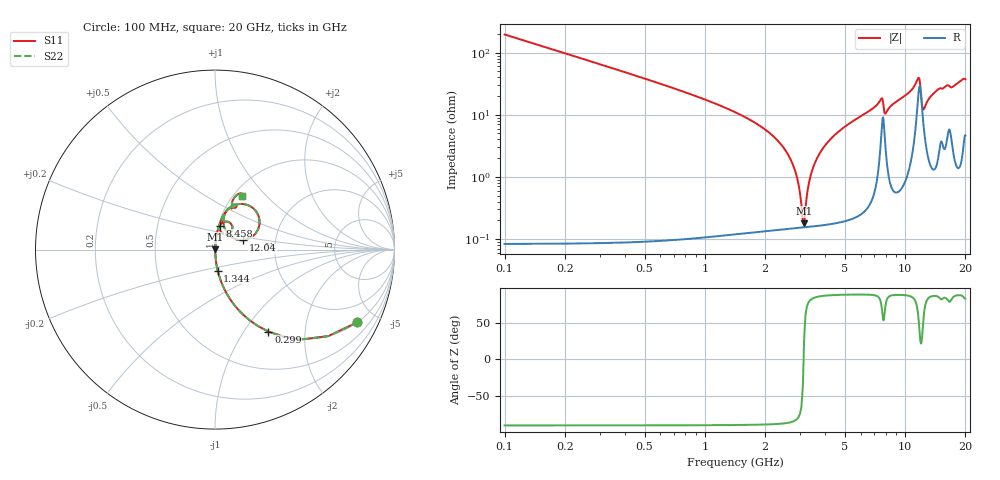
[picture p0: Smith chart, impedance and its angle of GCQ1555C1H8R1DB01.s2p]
!Murata Part Number: GCQ1555C1H8R1DB01
!These Parameters are Measured in Series Mode Connection
!Data Generated on Jan 08, 2026
!  o--ll--o
!Port1  Port2
!  o------o
!Operation Temp=25[degC], DC Bias Voltage=0[V]
!Freq. Start=100[MHz] Stop=20[GHz] 401[Steps]
# Hz S RI R 50
!Freq.(Hz) S11(Real) S11(Imag) S21(Real) S21(Imag) S12(Real) S12(Imag) S22(Real) S22(Imag)
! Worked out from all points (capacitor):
!   401 points, 100 MHz to 20 GHz, reference 50 ohm
!   read as one part in series: C = 8.1 pF near 199.5 MHz
!   lowest |Z| = 178 mohm at 3.135 GHz (marker M1)
!   series resonance near 3.113 GHz, so ESL is about 320 pH
!   S11 on the Smith chart (normalised r, x): 100 MHz: 1.00, -3.93; 299 MHz: 1.00, -1.30; 1.344 GHz: 1.00, -0.24; 8.458 GHz: 1.01, +0.27; 12.04 GHz: 1.37, +0.15; 20 GHz: 1.09, +0.74
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1e8  0.7938 -0.4043  0.2062 0.4043  0.2062 0.4043  0.7938 -0.4043
2.99e8  0.2979 -0.4567  0.7021 0.4567  0.7021 0.4567  0.2979 -0.4567
5.975e8  0.0918 -0.2873  0.9082 0.2873  0.9082 0.2873  0.0918 -0.2873
1.34375e9  0.0151 -0.117  0.9849 0.117  0.9849 0.117  0.0151 -0.117
2.5875e9  0.00199 -0.0235  0.998 0.0235  0.998 0.0235  0.00199 -0.0235
2.83625e9  0.00162 -0.0118  0.9984 0.0118  0.9984 0.0118  0.00162 -0.0118
3.03525e9  0.00152 -0.00319  0.9985 0.00319  0.9985 0.00319  0.00152 -0.00319
3.13475e9  0.00153 0.000904  0.9985 -0.000904  0.9985 -0.000904  0.00153 0.000904
3.43325e9  0.00174 0.0125  0.9983 -0.0125  0.9983 -0.0125  0.00174 0.0125
3.83125e9  0.00236 0.0267  0.9976 -0.0267  0.9976 -0.0267  0.00236 0.0267
4.42825e9  0.00391 0.0462  0.9961 -0.0462  0.9961 -0.0462  0.00391 0.0462
6.7665e9  0.0182 0.1182  0.9818 -0.1182  0.9818 -0.1182  0.0182 0.1182
7.61225e9  0.0736 0.155  0.9264 -0.155  0.9264 -0.155  0.0736 0.155
7.9605e9  0.041 0.0917  0.959 -0.0917  0.959 -0.0917  0.041 0.0917
8.458e9  0.0253 0.1321  0.9747 -0.1321  0.9747 -0.1321  0.0253 0.1321
1.005e10  0.048 0.1936  0.952 -0.1936  0.952 -0.1936  0.048 0.1936
1.159225e10  0.2143 0.229  0.7857 -0.229  0.7857 -0.229  0.2143 0.229
1.204e10  0.1585 0.053  0.8415 -0.053  0.8415 -0.053  0.1585 0.053
1.23385e10  0.0744 0.0849  0.9256 -0.0849  0.9256 -0.0849  0.0744 0.0849
1.338325e10  0.0498 0.182  0.9502 -0.182  0.9502 -0.182  0.0498 0.182
1.67165e10  0.1149 0.2336  0.8851 -0.2336  0.8851 -0.2336  0.1149 0.2336
2e10  0.1506 0.3004  0.8494 -0.3004  0.8494 -0.3004  0.1506 0.3004
